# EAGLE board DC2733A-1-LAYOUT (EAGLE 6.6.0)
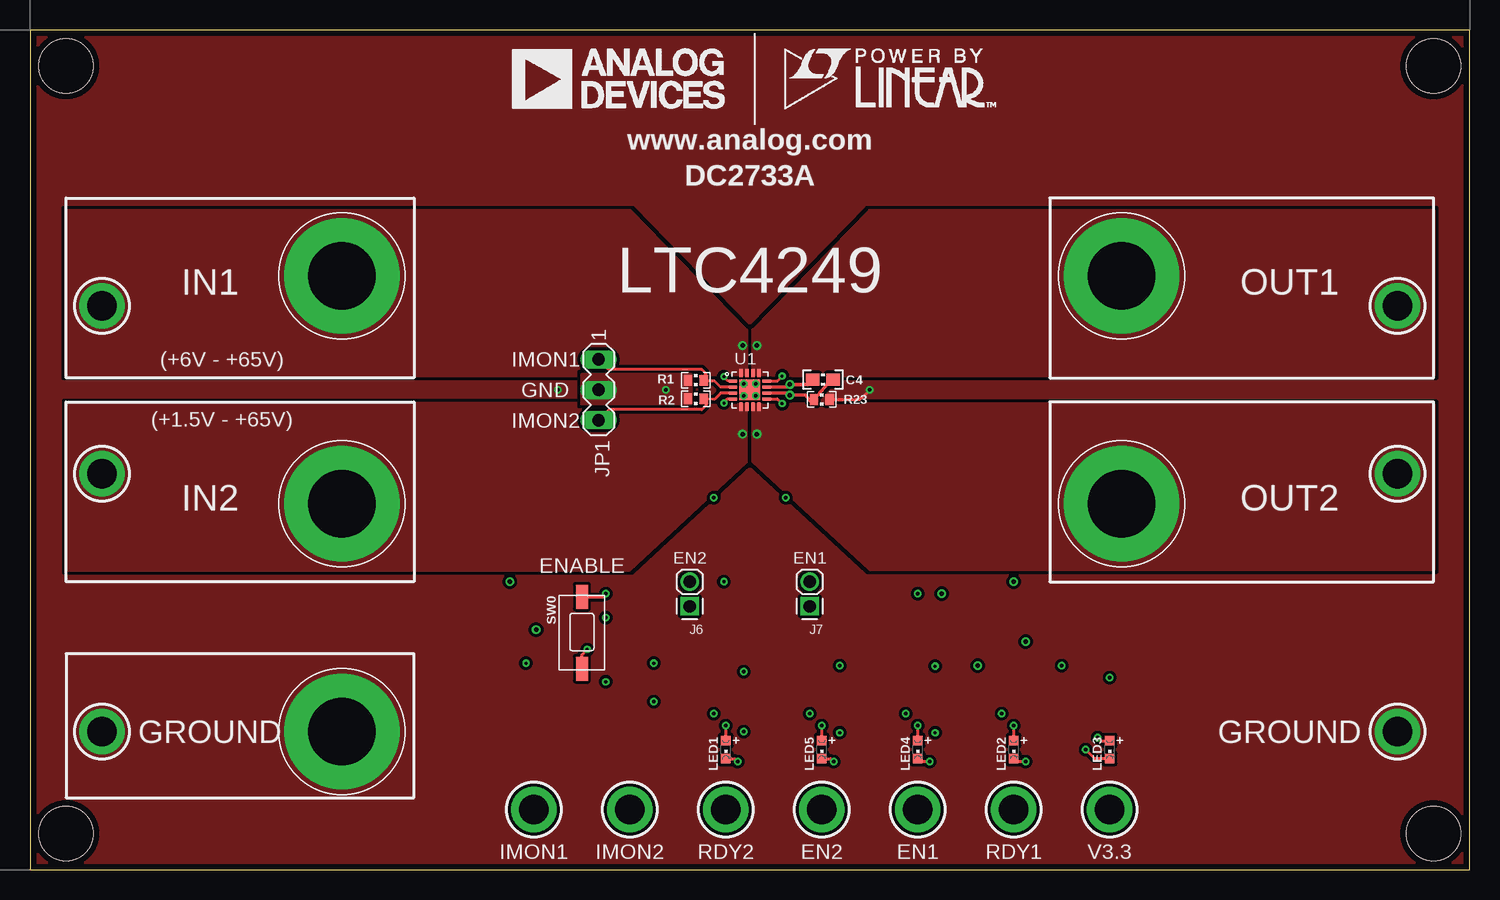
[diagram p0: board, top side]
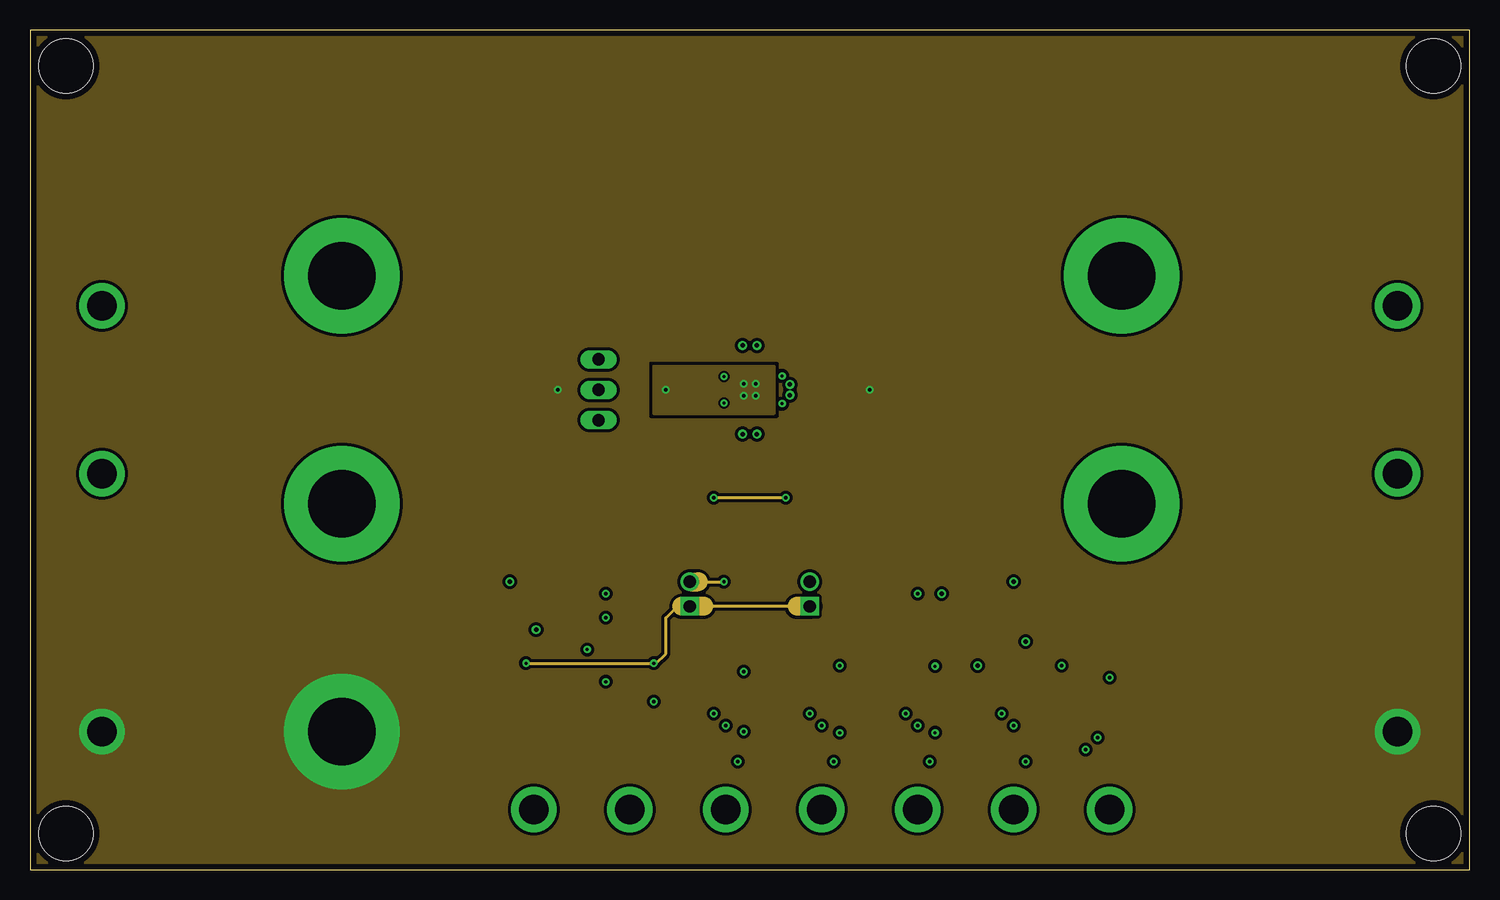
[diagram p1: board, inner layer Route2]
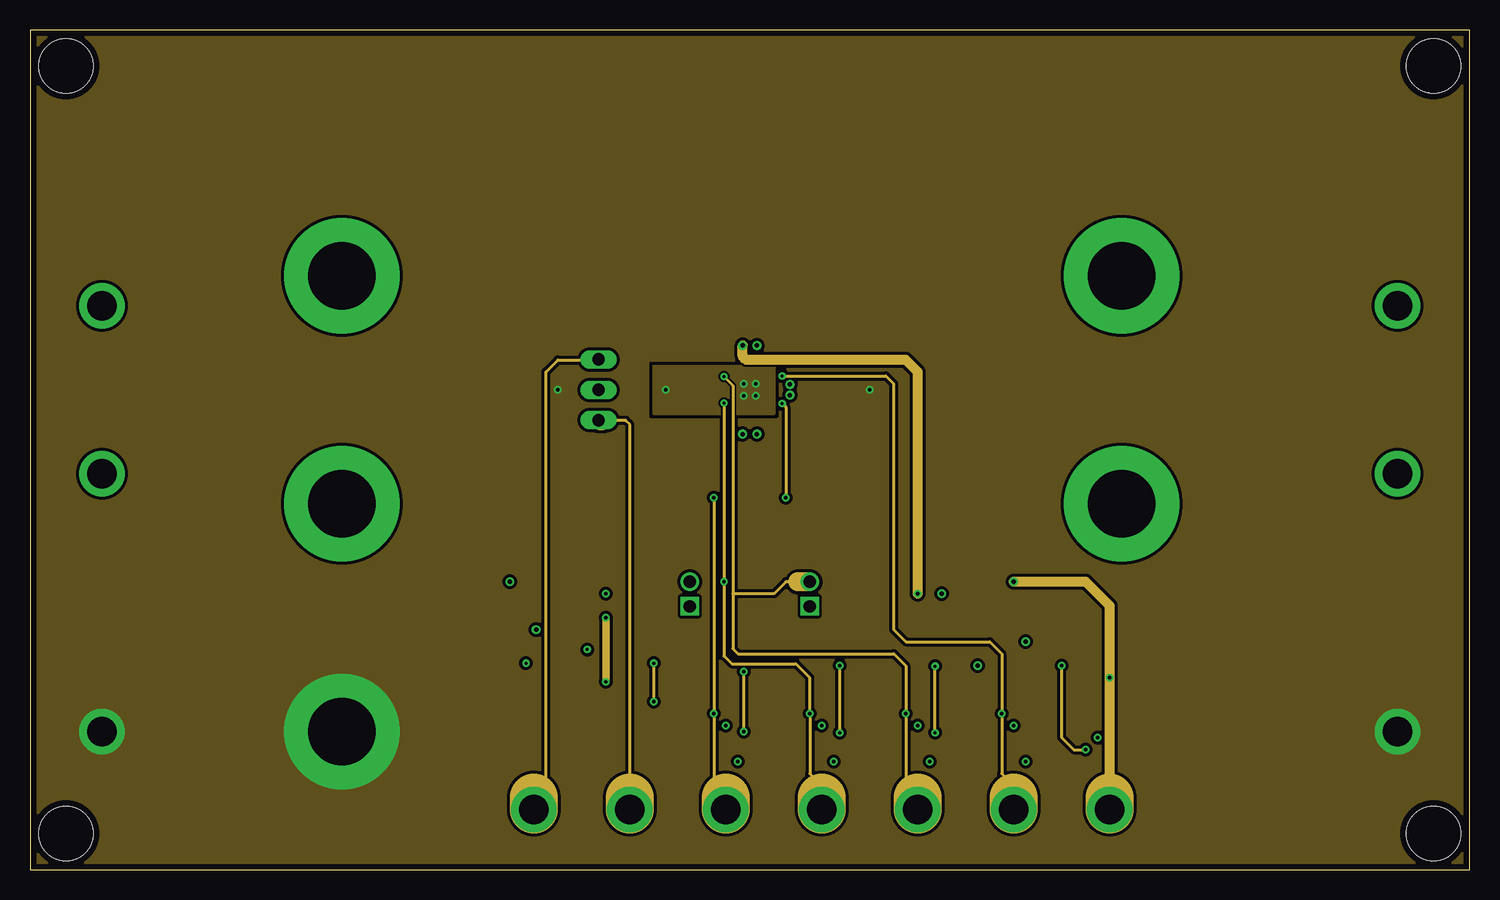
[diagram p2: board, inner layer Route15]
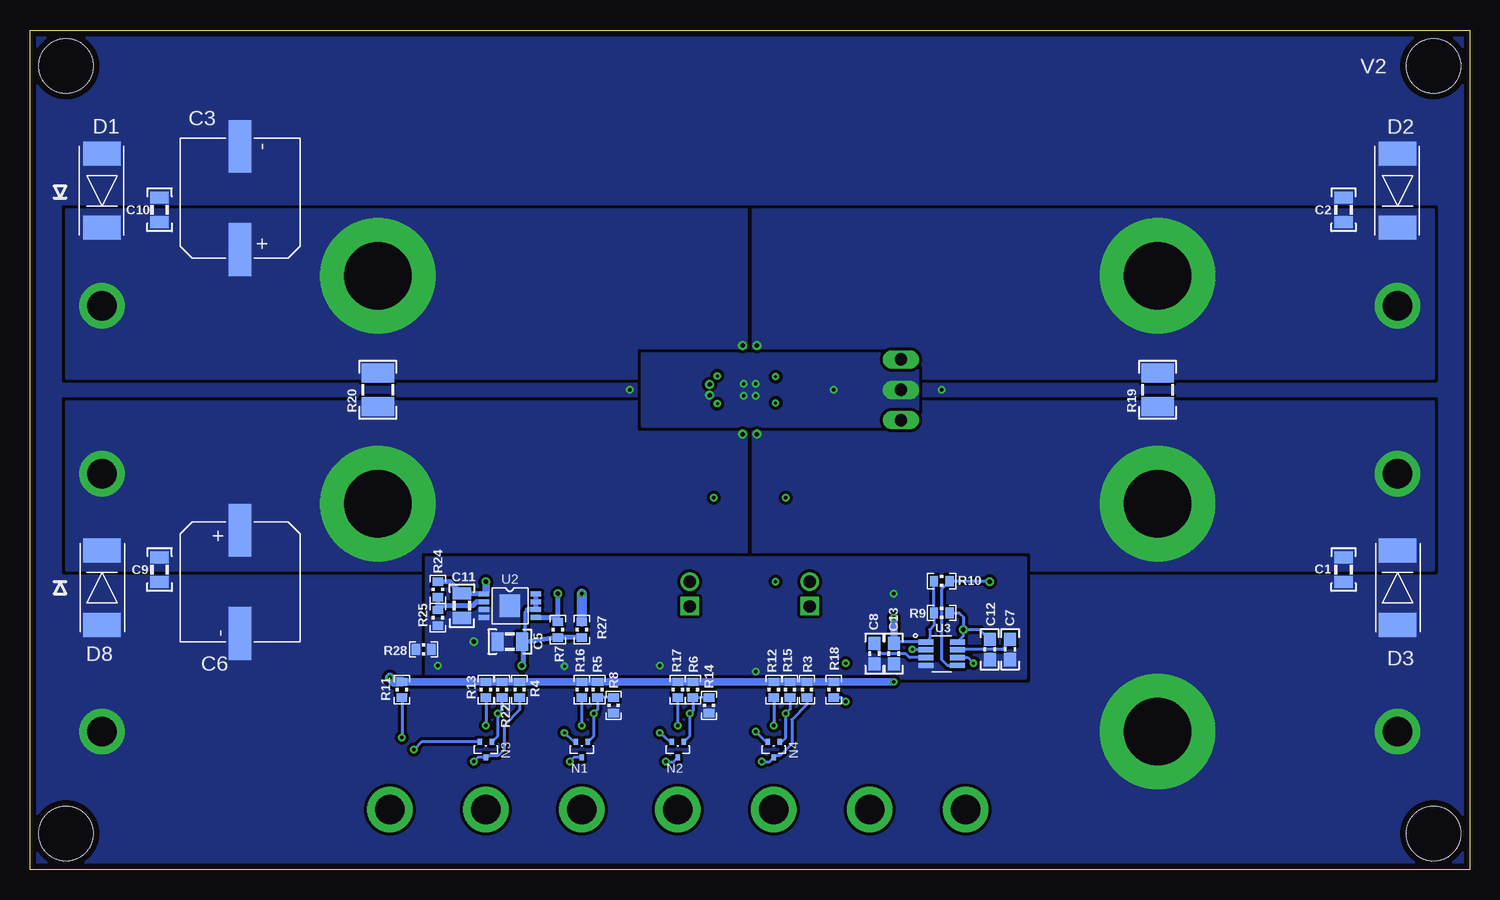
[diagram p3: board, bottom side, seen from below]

Size 120 x 70 mm. Coordinates in mm from the lower left corner, seen from the top.
Outline: 0,0 120,0 120,70 0,70 0,0
Copper layers (1+2*15+16): Top 0.07mm / dielectric 0.23mm / Route2 0.035mm / dielectric 1.01mm / Route15 0.035mm / dielectric 0.2mm / Bottom 0.07mm
Design rules "nicks-panel": minimum track width 6mil, minimum drill 10mil, track to track 6mil, track to pad 6mil, pad to pad 6mil, via to via 6mil, smd to smd 6mil, copper to edge 20mil, drill to drill 8mil, minimum pad ring 7mil, minimum via ring 7mil, stop-mask expansion 2.5mil, vias tented up to drill 14mil, thermal gap 10mil
Holes 4.5 mm at 3,3 117,3 117,67 3,67

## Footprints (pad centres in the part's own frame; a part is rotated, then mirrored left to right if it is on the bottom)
C0805_BOX = smd 1.016 x 1.524: 1 -1.016,0; 2 1.016,0
CAP-CAN = smd 4.4 x 1.9: P$1 4.3,0; P$2 -4.3,0
C0603_BOX = smd 1.1 x 1: 1 -0.85,0; 2 0.85,0
DO-214AB = smd 2 x 3.1: P$1 -3.09,0; P$2 3.09,0
BANANA = drill 5.588 pad 9.652: 1 0,0
1X02 = drill 1.016 square: 1 -2.05,0 | drill 1.016: 2 0,0
MA03-1 = drill 1.016 long: 1 -2.54,0; 2 0,0; 3 2.54,0
CHIPLED_0603 = smd 0.8 x 0.8: A 0,-0.75; C 0,0.75
SOT523-3 = smd 0.4 x 0.51: D 0,0.65; G -0.5,-0.65; S 0.5,-0.65
R0402_BOX = smd 0.7 x 0.9: 1 -0.65,0; 2 0.65,0
R1210_BOX = smd 1.6 x 2.7: 1 -1.4,0; 2 1.4,0
SWITCH_PTS635 = smd 2 x 1: SW1 -3,0; SW2 3,0
TP1 = drill 2.438 pad 3.81: TP 0,0
VIA = drill 0.381: 1 0,0
QFN-16-3X3 = smd 0.7 x 0.25: P$1 -1.4,0.75; P$2 -1.4,0.25; P$3 -1.4,-0.25; P$4 -1.4,-0.75; P$9 1.4,-0.75; P$10 1.4,-0.25; P$11 1.4,0.25; P$12 1.4,0.75 | smd 0.25 x 0.7: P$5 -0.75,-1.4; P$6 -0.25,-1.4; P$7 0.25,-1.4; P$8 0.75,-1.4; P$13 0.75,1.4; P$14 0.25,1.4; P$15 -0.25,1.4; P$16 -0.75,1.4 | smd 1.7 x 1.7: P$17 0,0
MS8E = smd 0.889 x 0.42: P$1 -2.171,0.975; P$2 -2.171,0.325; P$3 -2.171,-0.325; P$4 -2.171,-0.975; P$5 2.171,-0.975; P$6 2.171,-0.325; P$7 2.171,0.325; P$8 2.171,0.975 | smd 1.68 x 1.88: P$9 0,0
TSOT23-8 = smd 1.22 x 0.45: P1 -1.31,0.975; P2 -1.31,0.325; P3 -1.31,-0.325; P4 -1.31,-0.975; P5 1.31,-0.975; P6 1.31,-0.325; P7 1.31,0.325; P8 1.31,0.975

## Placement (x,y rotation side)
C1  1u  [C0805_BOX]  10.5,25 270 bottom
C2  1u  [C0805_BOX]  10.5,55 270 bottom
C3  DNI  [CAP-CAN]  102.5,56 270 bottom
C4  0.1u  [C0603_BOX]  66.1,40.85 180 top
C5  1u  [C0805_BOX]  80,19 0 bottom
C6  DNI  [CAP-CAN]  102.5,24 90 bottom
C7  DNI  [C0603_BOX]  38.3,18.35 270 bottom
C8  DNI  [C0603_BOX]  49.6,18 270 bottom
C9  1u/100V  [C0805_BOX]  109.2,25 270 bottom
C10  1u/100V  [C0805_BOX]  109.2,55 270 bottom
C11  2.2u  [C0805_BOX]  84,22 90 bottom
C12  0.01u  [C0603_BOX]  40,18.35 270 bottom
C13  0.1u  [C0603_BOX]  48,18 270 bottom
D1  SMCJXXA  [DO-214AB]  114,56.6 270 bottom
D2  SMCJXXA  [DO-214AB]  6,56.6 270 bottom
D3  SMCJXXA  [DO-214AB]  6,23.5 90 bottom
D8  SMCJXXA  [DO-214AB]  114,23.5 90 bottom
J1  BANANA  [BANANA]  26,49.5 0 top
J2  BANANA  [BANANA]  26,30.5 0 top
J3  BANANA  [BANANA]  91,30.5 0 top
J4  BANANA  [BANANA]  91,49.5 0 top
J5  BANANA  [BANANA]  26,11.5 0 top
J6  PINHD-1X2  [1X02]  55,24 90 top
J7  PINHD-1X2  [1X02]  65,24 90 top
JP1  [MA03-1]  47.4,40 270 top
LED1  LED-0603  [CHIPLED_0603]  58,10 180 top
LED2  LED-0603  [CHIPLED_0603]  82,10 180 top
LED3  LED-0603  [CHIPLED_0603]  90,10 180 top
LED4  LED-0603  [CHIPLED_0603]  74,10 180 top
LED5  LED-0603  [CHIPLED_0603]  66,10 180 top
N1  DMG1012T  [SOT523-3]  74,10 180 bottom
N2  DMG1012T  [SOT523-3]  66,10 180 bottom
N3  DMG1012T  [SOT523-3]  82,10 180 bottom
N4  DMG1012T  [SOT523-3]  58,10 180 bottom
R1  10k  [R0402_BOX]  55.5,40.8 0 top
R2  10k  [R0402_BOX]  55.5,39.25 0 top
R3  100k  [R0402_BOX]  55.23,15 90 bottom
R4  100k  [R0402_BOX]  79.2,15 90 bottom
R5  DNI  [R0402_BOX]  72.7,15 90 bottom
R6  DNI  [R0402_BOX]  64.75,15 90 bottom
R7  10k  [R0402_BOX]  76,20 270 bottom
R8  499k  [R0402_BOX]  71.35,13.7 270 bottom
R9  100k  [R0402_BOX]  44,21.4 0 bottom
R10  100k  [R0402_BOX]  44,24.05 0 bottom
R11  4.99k  [R0402_BOX]  89,15 90 bottom
R12  4.99k  [R0402_BOX]  58,15 90 bottom
R13  4.99k  [R0402_BOX]  82,15 270 bottom
R14  499k  [R0402_BOX]  63.4,13.7 90 bottom
R15  100k  [R0402_BOX]  56.65,15 90 bottom
R16  4.99k  [R0402_BOX]  74,15 90 bottom
R17  4.99k  [R0402_BOX]  66,15 90 bottom
R18  10k  [R0402_BOX]  53,15 90 bottom
R19  DNI  [R1210_BOX]  26,40 90 bottom
R20  DNI  [R1210_BOX]  91,40 90 bottom
R22  100k  [R0402_BOX]  80.65,15 90 bottom
R23  0  [R0402_BOX]  66,39.2 180 top
R24  15.8k  [R0402_BOX]  86,23.35 90 bottom
R25  10k  [R0402_BOX]  86,21 90 bottom
R27  0  [R0402_BOX]  74,20 270 bottom
R28  0  [R0402_BOX]  87.2,18.35 180 bottom
SW0  PTS635SL25SMTR LFS  [SWITCH_PTS635]  46,19.75 270 top
TP1  TESTPOINT_BIG  [TP1]  6,47 0 top
TP2  TESTPOINT_BIG  [TP1]  6,33 0 top
TP3  TESTPOINT_BIG  [TP1]  114,47 0 top
TP4  TESTPOINT_BIG  [TP1]  114,33 0 top
TP5  TESTPOINT  [VIA]  76,23 0 top
TP6  TESTPOINT_BIG  [TP1]  6,11.5 0 top
TP7  TESTPOINT_BIG  [TP1]  114,11.5 0 top
TP8  TESTPOINT  [VIA]  59.4,43.7 90 top
TP9  TESTPOINT  [VIA]  59.4,36.3 0 top
TP10  TESTPOINT  [VIA]  60.6,36.3 0 top
TP11  TESTPOINT  [VIA]  60.6,43.7 0 top
TP12  TESTPOINT  [VIA]  82,24 0 top
TP13  TESTPOINT  [VIA]  83,19 0 top
TP14  TESTPOINT  [VIA]  79,17 0 top
TP15  TESTPOINT  [VIA]  40,24 0 top
TP16  TESTPOINT  [VIA]  63.35,40.45 0 top
TP17  TESTPOINT  [VIA]  63.35,39.55 0 top
TP18  TESTPOINT  [VIA]  42.2,20 0 top
TP19  TESTPOINT_BIG  [TP1]  90,5 0 top
TP20  TESTPOINT_BIG  [TP1]  82,5 0 top
TP21  TESTPOINT_BIG  [TP1]  58,5 0 top
TP22  TESTPOINT_BIG  [TP1]  74,5 0 top
TP23  TESTPOINT_BIG  [TP1]  66,5 0 top
TP24  TESTPOINT_BIG  [TP1]  42,5 0 top
TP25  TESTPOINT_BIG  [TP1]  50,5 0 top
U1  LTC4249-16  [QFN-16-3X3]  60,40 0 top
U2  LT3010  [MS8E]  80,22 0 bottom
U3  LTC2954  [TSOT23-8]  44,18 0 bottom
U$3  [PBL-LOGO-700DPI]  40,62 0 top

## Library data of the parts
C1 C2 C4 C5 C7-C13 J1-J5 LED1-LED5 R1-R20 R22-R25 R27 R28 SW0 TP1-TP25 = kalin
C3 C6 D1-D3 D8 J6 J7 N1-N4 = nengerLib
JP1 = con-lstb; OC_FARNELL: unknown; OC_NEWARK: unknown
U1-U3 = LTC-DEVICES
U$3 = FOO

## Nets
+3V3: C11.2 C13.1 R3.2 R4.2 R5.2 R6.2 R9.1 R10.1 R11.2 R12.2 R13.1 R15.2 R16.2 R17.2 R18.2 R22.2 R24.2 TP12.1 TP19.TP U2.P$1 U3.P1
EN1: J7.2 N1.G R5.1 R8.1 TP22.TP U1.P$1
EN2: J6.2 N2.G R6.1 R14.2 TP23.TP U1.P$4
EN_PB: J6.1 J7.1 R18.1 U3.P6
GND: C4.1 JP1.2 R1.1 R2.1 R23.2 TP17.1 U1.P$10 U1.P$17
GND2: C5.1 C7.2 C8.2 C11.1 C12.2 C13.2 LED3.C N1.S N2.S N3.S N4.S R25.1 R28.1 SW0.SW1 TP13.1 U2.P$3 U2.P$4 U2.P$9 U3.P4
GROUND: C1.2 C2.1 C3.P$2 C6.P$2 C9.2 C10.1 D1.P$1 D2.P$1 D3.P$1 D8.P$1 J5.1 R8.2 R14.1 R23.1 R28.2 TP6.TP TP7.TP
IMON1: JP1.1 R1.2 TP24.TP U1.P$2
IMON2: JP1.3 R2.2 TP25.TP U1.P$3
IN1: C2.2 D2.P$2 J1.1 R19.2 R27.1 TP1.TP TP8.1 U1.P$15 U1.P$16
IN2: C1.1 D3.P$2 J2.1 R19.1 TP2.TP TP9.1 U1.P$5 U1.P$6
N$1: C4.2 TP16.1 U1.P$11
N$2: LED2.A R13.2
N$3: LED1.A R12.1
N$4: C8.1 U3.P3
N$5: C7.1 U3.P7
N$6: LED3.A R11.1
N$7: LED5.C N2.D
N$8: C12.1 R9.2 TP18.1 U3.P8
N$9: LED4.C N1.D
N$10: R24.1 R25.2 U2.P$2
N$11: R10.2 TP15.1 U3.P5
N$12: LED4.A R16.1
N$13: R7.1 TP5.1 U2.P$5
N$14: LED5.A R17.1
OUT1: C3.P$1 C10.2 D1.P$2 J4.1 R20.2 TP3.TP TP11.1 U1.P$13 U1.P$14
OUT2: C6.P$1 C9.1 D8.P$2 J3.1 R20.1 TP4.TP TP10.1 U1.P$7 U1.P$8
PB_EN: SW0.SW2 U3.P2
RDY1: N3.G R22.1 TP20.TP U1.P$12
RDY1B: LED2.C N3.D R4.1
RDY2: N4.G R15.1 TP21.TP U1.P$9
RDY2B: LED1.C N4.D R3.1
V1: C5.2 R7.2 R27.2 TP14.1 U2.P$6 U2.P$7 U2.P$8

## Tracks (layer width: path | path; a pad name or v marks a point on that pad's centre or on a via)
+3V3  (via drill 0.25)
  Route15 0.61: v48,15.65 v48,21
  Route15 0.813: 90,6 v90,16 90,22 88,24 TP12.1
  Route15 4: TP19.TP 90,6
  Bottom 0.254: 45.28,18.95 U3.P1 | U3.P1 47.88,18.98 C13.1 | U3.P1 45,19.29 45,20 44.65,20.35 R9.1 R10.1
  Bottom 0.406: R24.2 85,24 84.02,23.02 C11.2 83.96,22.98 U2.P$1 82,23.15
  Bottom 0.61: 82,23.15 TP12.1 | R11.2 R22.2 R13.1 R4.2 R16.2 R5.2 R17.2 R6.2 R12.2 R15.2 R3.2 R18.2 v48,15.65 | v48,21 C13.1
  Bottom 0.813: R11.2 89.65,15.65 v90,16
EN1  (via drill 0.25)
  Top 0.254: U1.P$1 58.2,40.75 v57.85,41.1
  Route15 0.254: v57.85,41.1 58.6,40.35 58.6,23 | 58.6,23 58.6,18.4 59,18 72,18 73,17 v73,13 73,6 TP22.TP | 64,24 63,24 62,23 58.6,23
  Route15 1.6: J7.2 64,24
  Route15 4: TP22.TP 74,6
  Bottom 0.254: N1.G 73,11.15 v73,13 72.7,13.3 R5.1 R8.1
EN2  (via drill 0.25)
  Top 0.254: U1.P$4 58.15,39.25 v57.85,38.9
  Route2 0.254: 55.7,24 v57.85,24
  Route2 1.6: J6.2 55.7,24
  Route15 0.254: v57.85,38.9 v57.85,24 57.85,17.8 58.5,17.15 63.85,17.15 65,16 v65,13 65,8 66,7 66,6
  Route15 4: TP23.TP 66,6
  Bottom 0.254: N2.G 65,11.15 v65,13 64.75,13.25 R6.1 R14.2
EN_PB  (via drill 0.25)
  Route2 0.254: 63.95,21.95 56.15,21.95 J6.1 54.95,22 54,22 53,21 53,18 52.2,17.2 v52,17.2 v41.35,17.2
  Route2 1.6: J7.1 63.95,21.95 | 56.15,21.95 54.35,21.95
  Route15 0.254: v52,14 v52,17.2
  Bottom 0.254: U3.P6 41.83,17.68 v41.35,17.2 | R18.1 52.35,14.35 v52,14
GND  (via drill 0.25)
  Top 0.254: R23.2 65.1,39 | C4.1 66.8,40.85 | U1.P$17 v59.5,39.5
  Top 0.305: U1.P$10 63.15,39.75 TP17.1 64.65,39.55 65.1,39 | 66.8,40.85 R23.2
  other vias: 59.5,40.5 53,40 60.5,40.5 60.5,39.5
  pour Bottom (isolate 0.254, no thermals): 46,43 69,43 69,37 46,37
  pour Top (no thermals): 55.1,41.3 55.1,38.8 46,38.8 46,41.3
  pour Route2: 52,42 62,42 62,38 52,38
  pour Route15: 52,42 62,42 62,38 52,38
GND2  (via drill 0.25)
  Top 0.254: SW0.SW1 47.75,22.75 v48,23 | LED3.C 88.75,9.25 v88,10
  Route15 0.254: v86,17 86,11 87,10 v88,10 | v75.45,11.4 v75.45,16.95 | v67.5,11.4 v67.5,17 | v59.5,11.5 v59.5,16.5
  Bottom 0.254: N1.S 74.65,10.65 v75.45,11.4 | N2.S 66.65,10.65 v67.5,11.4 | N4.S 58.65,10.65 v59.5,11.5 | N3.S 87.35,10.65 v88,10
  pour Bottom (isolate 0.254, no thermals): 37,26 87,26 87,16 37,16
GROUND  (via drill 0.25)
  Top 0.254: R23.1 69.2,39.2 v70,40
  other vias: 44,40
  pour Bottom (isolate 0.254, rank 3, no thermals): 0.5,69.5 119.5,69.5 119.5,0.5 0.5,0.5
  pour Top (isolate 0.254, rank 3, no thermals): 0.5,69.5 119.5,69.5 119.5,0.5 0.5,0.5
  pour Route15 (isolate 0.254, rank 2, no thermals): 0.5,69.5 119.5,69.5 119.5,0.5 0.5,0.5
  pour Route2 (isolate 0.254, rank 2, no thermals): 0.5,69.5 119.5,69.5 119.5,0.5 0.5,0.5
IMON1
  Top 0.254: U1.P$2 57.55,40.25 57.05,40.75 56.45,40.75 R1.2 56.35,41.35 56,41.7 48.24,41.7 JP1.1
  Route15 0.254: JP1.1 47.36,42.5 44,42.5 43,41.5 43,7 42,6
  Route15 4: TP24.TP 42,6
IMON2
  Top 0.254: U1.P$3 57.6,39.75 57.05,39.2 R2.2 56.35,38.7 56,38.35 48.29,38.35 JP1.3
  Route15 0.254: 50,6 50,37.1 49.65,37.45 47.8,37.45 JP1.3
  Route15 1.6: JP1.3 47.8,37.45
  Route15 4: TP25.TP 50,6
IN1  (via drill 0.25)
  Route15 0.813: v74,23 74,41.5 73,42.5 59.7,42.5 59.4,42.8 TP8.1
  Bottom 0.813: R27.1 v74,23
  pour Top (isolate 0.254, rank 2, no thermals): 59.74,41.15 3,41.15 3,55 50,55 59.74,45
  pour Bottom (isolate 0.254, rank 2, no thermals): 59.74,55 59.74,41 3,41 3,55
IN2
  pour Top (isolate 0.254, rank 2, no thermals): 59.74,38.85 3,38.85 3,25 50,25 59.74,34
  pour Bottom (isolate 0.254, rank 2, no thermals): 59.74,39 59.74,25 3,25 3,39
N$1
  Top 0.305: U1.P$11 63.15,40.25 TP16.1 64.85,40.45 C4.2
N$2  (via drill 0.25)
  Top 0.254: LED2.A v82,12
  Bottom 0.254: R13.2 v82,12
N$3  (via drill 0.25)
  Top 0.254: LED1.A v58,12
  Bottom 0.254: R12.1 v58,12
N$4
  Bottom 0.254: U3.P3 46.67,17.68 47,18 49,18 49.6,18.6 C8.1
N$5
  Bottom 0.254: U3.P7 42.66,18.35 38.95,18.35 38.3,19 C7.1
N$6  (via drill 0.25)
  Top 0.254: v89,11 89.25,10.75 LED3.A
  Bottom 0.254: R11.1 v89,11
N$7  (via drill 0.25)
  Top 0.254: LED5.C 66.75,9.25 v67,9
  Bottom 0.254: v67,9 66.35,9 N2.D
N$8
  Bottom 0.254: R9.2 42.55,21.4 42.2,21.05 TP18.1 | U3.P8 42.2,19.46 TP18.1 | C12.1 40.8,20 TP18.1
N$9  (via drill 0.25)
  Top 0.254: v75,9 74.25,9 LED4.C
  Bottom 0.254: N1.D 74.65,9.35 v75,9
N$10
  Bottom 0.406: R24.1 R25.2 85.65,22 83.1,22 82.78,22.32 U2.P$2
N$11
  Bottom 0.254: U3.P5 42.66,17 43.5,17 44,17.5 44,23.4 R10.2 40.05,24.05 TP15.1
N$12  (via drill 0.25)
  Top 0.254: LED4.A v74,12
  Bottom 0.254: v74,12 R16.1
N$13
  Bottom 0.406: U2.P$5 76.05,21.02 R7.1 TP5.1
N$14  (via drill 0.25)
  Top 0.254: LED5.A v66,12
  Bottom 0.254: v66,12 R17.1
OUT1
  pour Top (isolate 0.254, rank 2, no thermals): 117,41.15 60.26,41.15 60.26,45 70,55 117,55
  pour Bottom (isolate 0.254, rank 2, no thermals): 117,55 117,41 60.26,41 60.26,55
OUT2
  pour Top (isolate 0.254, rank 2, no thermals): 60.26,38.85 117,38.85 117,25 70,25 60.26,34
  pour Bottom (isolate 0.254, rank 2, no thermals): 117,39 117,25 60.26,25 60.26,39
PB_EN  (via drill 0.25)
  Top 0.254: SW0.SW2 46,17.9 v46.45,18.35
  Bottom 0.254: U3.P2 46.38,18.32 v46.45,18.35
RDY1  (via drill 0.25)
  Top 0.254: U1.P$12 62.3,40.75 v62.7,41.15
  Route15 0.254: v62.7,41.15 71.35,41.15 72,40.5 72,20 73,19 80,19 81,18 v81,13 81,8 82,7 82,6
  Route15 4: TP20.TP 82,6
  Bottom 0.254: N3.G 81,11.15 v81,13 80.65,13.35 R22.1
RDY1B  (via drill 0.25)
  Top 0.254: v83,9 82.25,9 LED2.C
  Bottom 0.254: v83,9 82.65,9.35 N3.D LED2.C 81.75,9.5 81,9.5 80.5,10 80.5,12 79.2,13.3 R4.1
RDY2  (via drill 0.25)
  Top 0.254: U1.P$9 62.3,39.25 v62.7,38.85
  Route2 0.254: v63,31 v57,31
  Route15 0.254: v62.7,38.85 63,38.55 v63,31 | v57,31 v57,13 57,6
  Route15 0.406: 57,6 TP21.TP
  Route15 4: TP21.TP 58,6
  Bottom 0.254: N4.G 57.35,10.65 57,11 v57,13 56.65,13.35 R15.1
RDY2B  (via drill 0.25)
  Top 0.254: LED1.C 58.75,9.25 v59,9
  Bottom 0.254: R3.1 55.23,13.77 56.5,12.5 56.5,10.5 57.5,9.5 57.85,9.5 N4.D 58.35,9 v59,9
V1
  Bottom 0.305: 78.53,21.68 78.75,21.45 78.75,19.23
  Bottom 0.406: R27.2 R7.2 78.91,18.92 | 78.91,18.92 C5.2 78.75,19.23 | 78.53,21.68 U2.P$6 U2.P$7 U2.P$8 | 78.91,18.92 78.91,17.09 TP14.1

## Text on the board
tNames: www.analog.com | DC2733A | LTC4249 | IN1 | OUT1 | (+6V - +65V) | IMON1 | GND | (+1.5V - +65V) | IMON2 | IN2 | OUT2 | EN2 | EN1 | ENABLE | GROUND | GROUND | IMON1 | IMON2 | RDY2 | EN2 | EN1 | RDY1 | V3.3
bNames: V2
